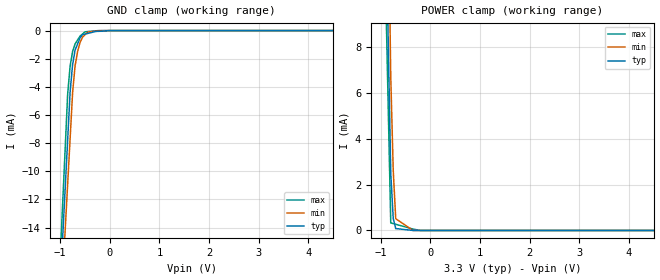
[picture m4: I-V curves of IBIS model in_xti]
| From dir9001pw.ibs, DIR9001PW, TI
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[Model] in_xti
Model_type Input
Vinl = 990.000mV
Vinh = 2.31000V
C_comp 546.0fF   546.0fF   546.0fF
| variable typ   min   max
[Voltage Range] 3.30000V 2.70000V 3.60000V
[POWER Clamp Reference] 3.30000V 2.70000V 3.60000V
[GND Clamp Reference] 0.00000V 0.00000V 0.00000V
[Temperature Range]   25   85   -40
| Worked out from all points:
|   GND clamp passes 1 mA (typ) near -0.66 V on its own axis
|   POWER clamp passes 1 mA (typ) near -0.76 V on its own axis
[GND Clamp]
-3.3V     -176.5mA   -170.9mA   -194.1mA
-850mV    -7.794mA   -10.93mA   -4.531mA
-800mV    -4.351mA   -7.665mA   -2.509mA
-750mV    -2.413mA   -4.401mA   -1.487mA
-700mV    -1.39mA    -2.502mA   -950.4uA
-650mV    -953.9uA   -1.497mA   -671.6uA
-600mV    -517.6uA   -844.2uA   -392.9uA
-550mV    -293.2uA   -464.8uA   -240.2uA
-500mV    -250.2uA   -288.9uA   -87.46uA
-450mV    -207.2uA   -113uA     -71.2uA
-225mV    -55.95uA   -5.91uA    -5.821uA
6.6V      0A         0A         0A
[POWER Clamp]
-3.3V     283.2mA    392.4mA    274.6mA
-1.1V     36.19mA    52.99mA    30mA
-800mV    2.505mA    6.71mA     331.5uA
-750mV    518.7uA    2.625mA    301.4uA
-700mV    82.76uA    514.7uA    271.3uA
-350mV    0A         0A         60.28uA
-200mV    0A         0A         0A
6.6V      0A         0A         0A
